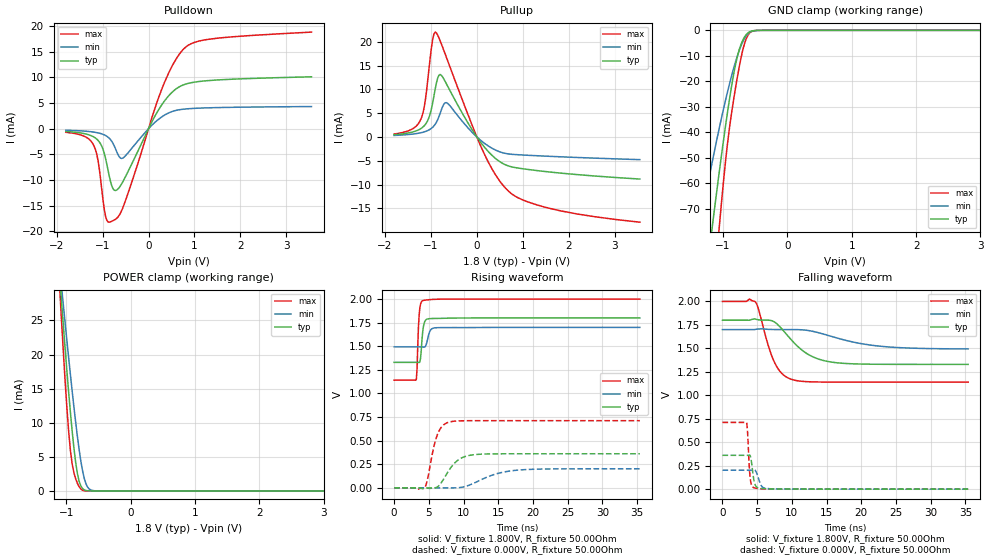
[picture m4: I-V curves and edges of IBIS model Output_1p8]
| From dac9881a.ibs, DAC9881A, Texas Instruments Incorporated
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|   Output_1p8 MODEL
[Model]   Output_1p8
Model_type   3-state
| Signals
Cref = 4.5pF   |Timing specification test load capacitance value
Rref = 5000Ohm
Vref = 2.5V
Vmeas = 0.9V
| variable   typ   min   max
|Output tri-stated
C_comp   4.029pF   4.685pF   3.174pF
|Output high
|C_comp   5.826pF   6.365pF   5.210pF
|Output low
|C_comp   7.717pF   6.616pF   7.033pF
| Junction Temperature (Ambient temp is 25C typ, 105C min,  -40C max)
[Temperature Range]   27   105   -40
[Voltage Range]   1.8V   1.7V   2.0V
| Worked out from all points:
|   slope of the pulldown table from 0 to 0.27 V, typ, clamps not added: 61.1 ohm
|   slope of the pullup table from 0 to 0.27 V, typ, clamps not added: 82.1 ohm
|   GND clamp passes 1 mA (typ) near -0.61 V on its own axis
|   POWER clamp passes 1 mA (typ) near -0.79 V on its own axis
|   falling waveform, V_fixture 1.800V, R_fixture 50.00Ohm: 20-80 % time 4.08ns typ, 7.08ns min, 2.25ns max; typ from 1.8 V to 1.33 V
|   rising waveform, V_fixture 1.800V, R_fixture 50.00Ohm: 20-80 % time 348ps typ, 461ps min, 278ps max; typ from 1.33 V to 1.8 V
|   rising waveform, V_fixture 0.000V, R_fixture 50.00Ohm: 20-80 % time 2.16ns typ, 4.22ns min, 1.31ns max; typ from 0 V to 0.361 V
|   falling waveform, V_fixture 0.000V, R_fixture 50.00Ohm: 20-80 % time 416ps typ, 597ps min, 319ps max; typ from 0.361 V to 0 V
[Pulldown]
|   Voltage   I(typ)   I(min)   I(max)
-1.8V     -529.4uA   -296.3uA   -697.8uA
-1.206V   -1.538mA   -643.6uA   -3.019mA
-1.098V   -2.281mA   -813.4uA   -6.242mA
-936mV    -5.764mA   -1.318mA   -17.05mA
-828mV    -10.26mA   -2.118mA   -18.17mA
-720mV    -12.06mA   -3.892mA   -17.67mA
-558mV    -10.32mA   -5.724mA   -15.39mA
279mV     4.54mA     2.247mA    7.496mA
522mV     7.192mA    3.381mA    12.37mA
765mV     8.577mA    3.816mA    15.57mA
1.278V    9.375mA    4.074mA    17.41mA
3.546V    10.13mA    4.326mA    18.86mA
[GND Clamp]
|   Voltage   I(typ)   I(min)   I(max)
-1.8V     -216.4mA   -140.7mA   -308mA
-1.368V   -119.3mA   -77.83mA   -170.9mA
-1.179V   -79.44mA   -53.01mA   -112.6mA
-1.152V   -73.95mA   -49.64mA   -104.5mA
-1.071V   -57.9mA    -39.83mA   -80.69mA
-1.044V   -52.71mA   -36.68mA   -73.05mA
-963mV    -37.77mA   -27.6mA    -51.74mA
-909mV    -28.49mA   -21.95mA   -39.96mA
-801mV    -12.86mA   -11.94mA   -21.82mA
-693mV    -3.839mA   -4.477mA   -7.668mA
-585mV    -545.3uA   -771.3uA   -1mA
3.546V    0A         0A         0A
[Pullup]
|   Voltage   I(typ)   I(min)   I(max)
-1.8V     460.9uA    312.6uA    613.6uA
-1.206V   1.841mA    914.7uA    4.03mA
-1.125V   2.577mA    1.135mA    7.451mA
-1.044V   4.031mA    1.471mA    14.16mA
-963mV    7.106mA    2.03mA     20.41mA
-909mV    9.955mA    2.641mA    22.05mA
-801mV    13.13mA    4.92mA     20.25mA
-666mV    11.23mA    7.217mA    16.82mA
117mV     -1.558mA   -972.1uA   -2.632mA
684mV     -6.085mA   -3.565mA   -11.35mA
1.575V    -7.357mA   -4.067mA   -14.99mA
3.546V    -8.849mA   -4.769mA   -17.92mA
[POWER Clamp]
|   Voltage   I(typ)   I(min)   I(max)
-1.8V     120.1mA    102.1mA    142.5mA
-1.098V   30.71mA    32.14mA    28.7mA
-1.071V   27.24mA    29.52mA    24.22mA
-1.044V   23.84mA    26.93mA    19.87mA
-990mV    17.33mA    21.84mA    11.89mA
-936mV    11.36mA    16.91mA    5.8mA
-882mV    6.202mA    12.22mA    2.631mA
-828mV    2.499mA    7.922mA    1.098mA
-747mV    328.9uA    2.866mA    95.82uA
-666mV    22.13uA    497.6uA    3.786uA
-558mV    606.9nA    22.08uA    70.11nA
3.546V    0A         0A         0A
[Ramp]
R_load = 50.00Ohm
|   typ   min   max
dV/dt_r   216.428mV/2.164ns   120.995mV/4.211ns   426.792mV/1.314ns
dV/dt_f   282.349mV/4.073ns   123.695mV/7.075ns   515.688mV/2.248ns
[Falling Waveform]
V_fixture = 1.800V
V_fixture_min = 1.700V
V_fixture_max = 2.000V
R_fixture = 50.00Ohm
|   Time   V(typ)   V(min)   V(max)
0s        1.8V       1.7V       2V
3.9ns     1.8V       1.7V       2.025V
4.8ns     1.81V      1.703V     1.99V
7.4ns     1.785V     1.701V     1.366V
8.5ns     1.712V     1.7V       1.237V
9.9ns     1.592V     1.7V       1.171V
12.5ns    1.429V     1.688V     1.144V
15.7ns    1.354V     1.627V     1.141V
23.2ns    1.33V      1.519V     1.14V
35.4ns    1.329V     1.494V     1.14V
[Rising Waveform]
V_fixture = 1.800V
V_fixture_min = 1.700V
V_fixture_max = 2.000V
R_fixture = 50.00Ohm
|   Time   V(typ)   V(min)   V(max)
0s        1.329V     1.494V     1.14V
3.2ns     1.329V     1.494V     1.151V
3.3ns     1.33V      1.494V     1.259V
3.5ns     1.329V     1.494V     1.699V
3.6ns     1.327V     1.494V     1.828V
3.8ns     1.37V      1.494V     1.944V
4.2ns     1.7V       1.492V     1.985V
4.6ns     1.782V     1.514V     1.99V
5.9ns     1.795V     1.695V     1.997V
35.4ns    1.8V       1.7V       2V
[Rising Waveform]
V_fixture = 0.000V
V_fixture_min = 0.000V
V_fixture_max = 0.000V
R_fixture = 50.00Ohm
|   Time   V(typ)   V(min)   V(max)
0s        13.4uV     21.78uV    1.803uV
4.4ns     -4.856mV   -169.2uV   3.306mV
4.8ns     -2.078mV   -3.772mV   87.93mV
5.6ns     -1.956mV   -2.769mV   394.2mV
6.2ns     8.103mV    -913.5uV   556.9mV
7.9ns     185.6mV    -843.7uV   696mV
9.6ns     311.8mV    3.922mV    709.8mV
11.9ns    353.5mV    63.52mV    711.2mV
18.1ns    360.6mV    189mV      711.3mV
35.4ns    360.7mV    201.7mV    711.3mV
[Falling Waveform]
V_fixture = 0.000V
V_fixture_min = 0.000V
V_fixture_max = 0.000V
R_fixture = 50.00Ohm
|   Time   V(typ)   V(min)   V(max)
0s        360.7mV    201.7mV    711.3mV
3.5ns     360.5mV    201.6mV    702.7mV
3.6ns     360.4mV    201.6mV    630.3mV
3.8ns     362.1mV    201.5mV    320.8mV
4ns       356.3mV    201.4mV    112.5mV
4.2ns     278.1mV    201.7mV    40.78mV
4.6ns     70.3mV     205mV      13.3mV
5.6ns     7.373mV    36.85mV    3.266mV
6.5ns     4.335mV    6.27mV     1.321mV
35.4ns    13.4uV     21.78uV    1.803uV
